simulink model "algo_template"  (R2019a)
settings: configuration reference "configurationSettings" (kept in a data dictionary, not in this file)
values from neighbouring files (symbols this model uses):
  Value = mystruct.(myfield)    [SCDsignal_struct_to_bus.m]
undefined symbols (not defined in the file or in its folder): algo_template_fp, algo_template_tp, ProductionState, QualityTag, signal1, signal2

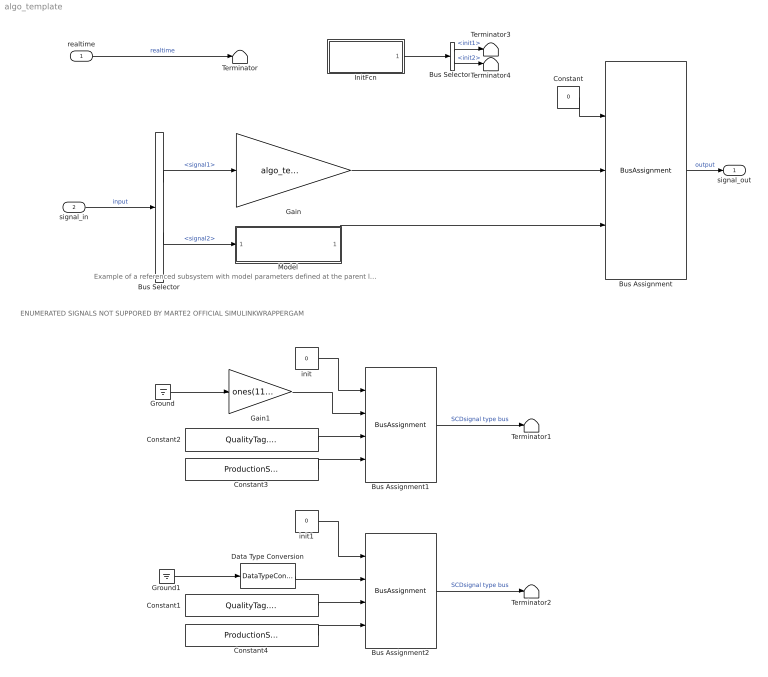
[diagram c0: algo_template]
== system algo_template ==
  note: ENUMERATED SIGNALS NOT SUPPORED BY MARTE2 OFFICIAL SIMULINKWRAPPERGAM
  note: Example of a referenced subsystem with model parameters defined at the parent level
  realtime : Inport  OutDataTypeStr=single  PortDimensions=1  SampleTime=algo_template_fp.timing.dt  Interpolate=off
  signal_in : Inport  Port=2  OutDataTypeStr=Bus: algo_template_inBus  PortDimensions=1  Interpolate=off
  Bus Assignment : BusAssignment  AssignedSignals=signal1,signal2
  Bus Assignment1 : BusAssignment  AssignedSignals=Value,QualityTag,ProductionState
  Bus Assignment2 : BusAssignment  AssignedSignals=Value,QualityTag,ProductionState
  Bus Selector : BusSelector  OutputSignals=signal1,signal2
  Bus Selector1 : BusSelector  OutputSignals=init1,init2
  Constant : Constant  Value=0  OutDataTypeStr=Bus: algo_template_outBus
  Constant1 : Constant  Value=QualityTag.INVALID  OutDataTypeStr=Enum: QualityTag
  Constant2 : Constant  Value=QualityTag.GOOD  OutDataTypeStr=Enum: QualityTag
  Constant3 : Constant  Value=ProductionState.RUNNING  OutDataTypeStr=Enum: ProductionState
  Constant4 : Constant  Value=ProductionState.OUTDATED  OutDataTypeStr=Enum: ProductionState
  Data Type Conversion : DataTypeConversion  Commented=through  OutDataTypeStr=int32
  Gain : Gain  Gain=algo_template_tp.gain
  Gain1 : Gain  Gain=ones(11,1)
  Ground : Ground
  Ground1 : Ground
  InitFcn : Subsystem  TreatAsAtomicUnit=on
  Model : ModelReference  ModelNameDialog=algo_template_referenced.slx  ParameterArgumentNames=TP  ParameterArgumentValues=algo_template_tp.refmodel  UsingDefaultArgumentValue=0  SimulationMode=Normal  ModelReferenceVersion=1.15
  Terminator{,1..4} (5 alike) : Terminator
  init : Constant  Value=0  OutDataTypeStr=Bus: SCDBus_single_11_Vector
  init1 : Constant  Value=0  OutDataTypeStr=Bus: SCDBus_int32_Scalar
  signal_out : Outport  OutDataTypeStr=Bus: algo_template_outBus
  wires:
  signal_in/1 -> Bus Selector/1  "input"
  Bus Selector/1 -> Gain/1  "<signal1>"
  Constant/1 -> Bus Assignment/1
  realtime/1 -> Terminator/1  "realtime"
  Bus Assignment/1 -> signal_out/1  "output"
  init/1 -> Bus Assignment1/1
  Bus Assignment1/1 -> Terminator1/1  "SCDsignal type bus"
  Constant2/1 -> Bus Assignment1/3
  Constant3/1 -> Bus Assignment1/4
  Gain1/1 -> Bus Assignment1/2
  init1/1 -> Bus Assignment2/1
  Data Type Conversion/1 -> Bus Assignment2/2
  Constant1/1 -> Bus Assignment2/3
  Constant4/1 -> Bus Assignment2/4
  Bus Assignment2/1 -> Terminator2/1  "SCDsignal type bus"
  Model/1 -> Bus Assignment/3
  Ground1/1 -> Data Type Conversion/1
  Ground/1 -> Gain1/1
  Gain/1 -> Bus Assignment/2
  Bus Selector/2 -> Model/1  "<signal2>"
  InitFcn/1(InitOut) -> Bus Selector1/1
  Bus Selector1/2 -> Terminator4/1  "<init2>"
  Bus Selector1/1 -> Terminator3/1  "<init1>"

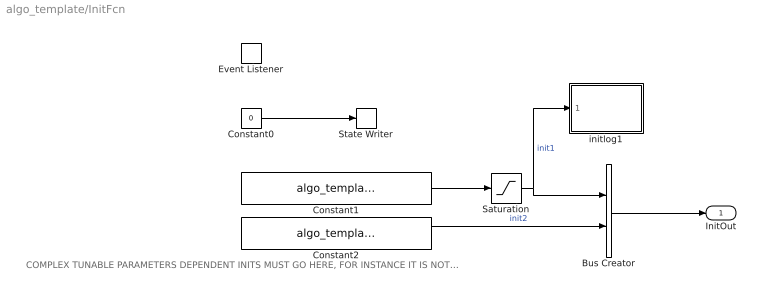
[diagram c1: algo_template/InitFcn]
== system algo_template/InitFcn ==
  note: COMPLEX TUNABLE PARAMETERS DEPENDENT INITS MUST GO HERE, FOR INSTANCE IT IS NOT POSSIBLE TO REFER TO A TUNABLE PARAMETER VIA DIRECT INDEXING IN MODEL DIALOG, THE VALUE MUST BE EXTRACTED HERE
  Bus Creator : BusCreator  Inputs=2
  Constant0 : Constant  Commented=on  Value=0
  Constant1 : Constant  Value=algo_template_tp.gain  OutDataTypeStr=single
  Constant2 : Constant  Value=algo_template_tp.rowvect(1)  OutDataTypeStr=int32
  Event Listener : EventListener  DisableCoverage=on  EventName=reset
  Saturation : Saturate
  State Writer : StateWriter  Commented=on
  initlog1 : MATLAB Function  TreatAsAtomicUnit=on
  InitOut : Outport  OutDataTypeStr=Bus: algo_template_init1
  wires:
  Constant0/1 -> State Writer/1
  Bus Creator/1 -> InitOut/1
  Constant1/1 -> Saturation/1
  Constant2/1 -> Bus Creator/2  "init2"
  Saturation/1 -> initlog1/1(u), Bus Creator/1  "init1"

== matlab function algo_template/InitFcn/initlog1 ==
function fcn(u)

fprintf('par value is %f',u);
